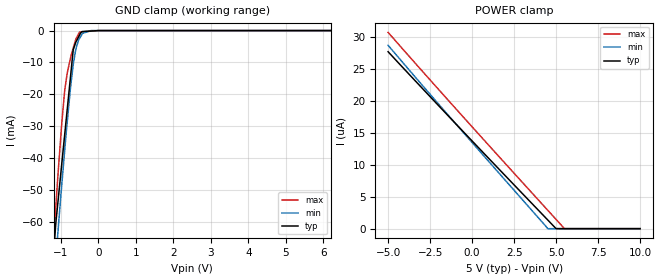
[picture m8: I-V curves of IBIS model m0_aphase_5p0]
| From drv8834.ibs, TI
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|   m0_aphase_5p0 Model
[Model]   m0_aphase_5p0
Model_type   Input
Vinl = 0.7
Vinh = 2
|   typ   min   max
|   (nom PVT)   (fast PVT)   (slow PVT)
|C_comp from frequency sweep method (F=250KHz)
|Average
|C_comp   2.902e-12   2.690e-12   3.123e-12
|C_comp from LC tank measurement(L=1nH)
|Average
|Resonant Frequency(Hz)   4.390e+09   4.450e+09   4.310e+09
 C_comp   1.316e-12   1.280e-12   1.365e-12
| Where nom  PVT is Nominal Process, 5V, 27C
|   Fast PVT is Strong Process,  5.5V, -40C
|   Slow PVT is Weak Process,   4.5V, 125C
[Voltage Range]   5   4.5   5.5
|Ambient Temperature   25   150   -40
|Junction Temperature
[Temperature Range]   27   125   -40
[Power Clamp Reference]   5   4.5   5.5
[GND Clamp Reference]   0   0   0
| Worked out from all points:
|   GND clamp passes 1 mA (typ) near -0.49 V on its own axis
[GND Clamp]
|   Voltage   I(typ)   I(min)   I(max)
-5V       -796.6mA   -746.9mA   -837.8mA
-1.216V   -73.1mA    -83.06mA   -68.39mA
-1.179V   -67.02mA   -77.42mA   -62.09mA
-1.14V    -60.52mA   -71.68mA   -55.36mA
-1.078V   -53.26mA   -62.54mA   -44.66mA
-907.5mV  -33.29mA   -38.36mA   -19.47mA
-836mV    -24.92mA   -28.92mA   -13.44mA
-675mV    -6.061mA   -10.76mA   -5.499mA
-603mV    -3.588mA   -5.766mA   -2.644mA
-506mV    -1.427mA   -2.475mA   -477.7uA
-202.5mV  -140.8uA   -11.29uA   -191.2uA
10V       0A         0A         0A
[POWER Clamp]
|   Voltage   I(typ)   I(min)   I(max)
-5V       27.65uA    28.65uA    30.67uA
-907.5mV  16.21uA    16.19uA    18.56uA
4.495V    1.379uA    15.62nA    2.896uA
4.995V    13.56nA    0A         1.456uA
5.505V    0A         0A         0A
10V       0A         0A         0A
